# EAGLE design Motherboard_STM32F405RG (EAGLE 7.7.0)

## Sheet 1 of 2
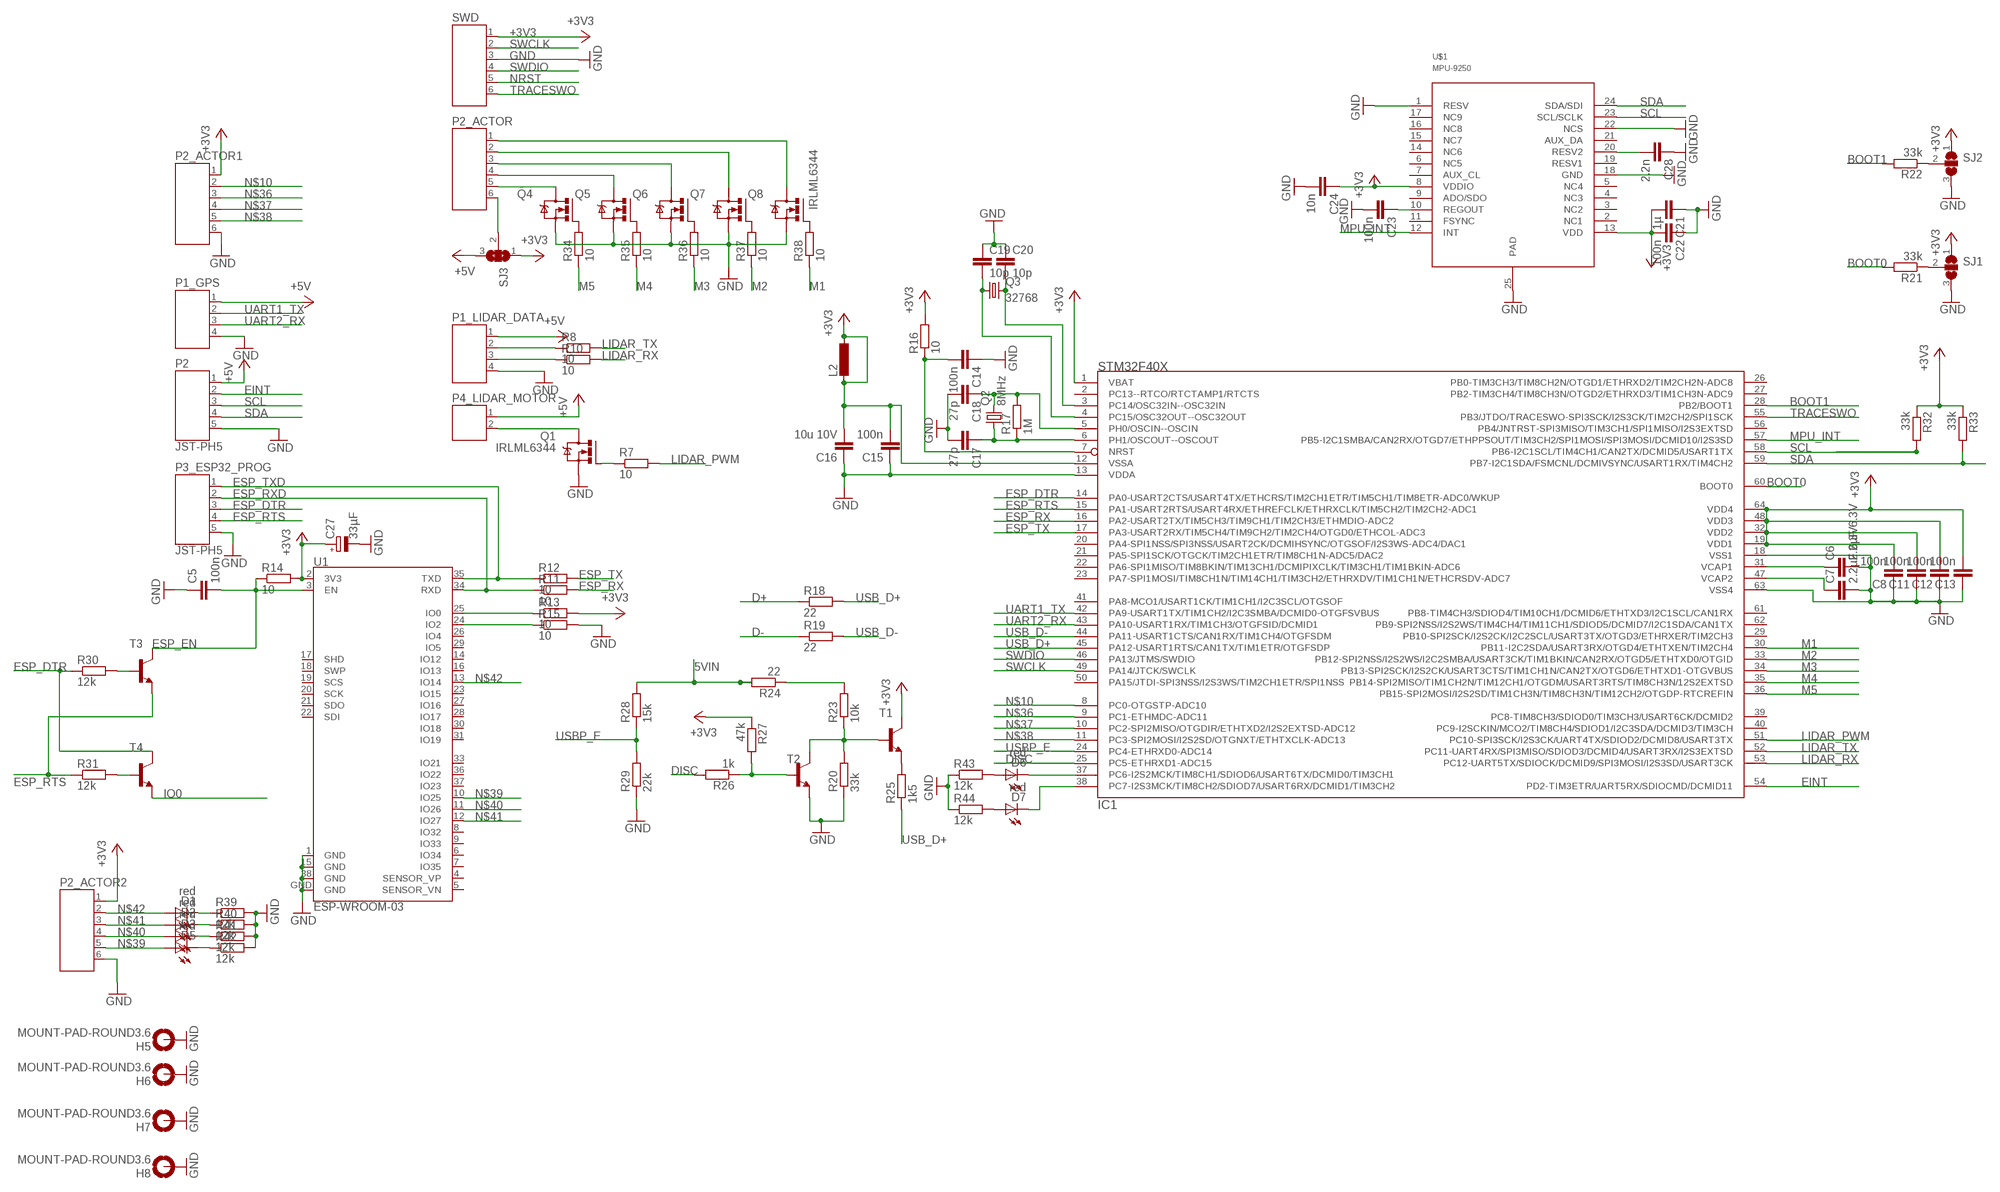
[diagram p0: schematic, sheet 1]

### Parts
C5  100n  C-EUC0603  [C0603]
C6  2.2µF 6.3V  C-EUC0603  [C0603]
C7  2.2µF 6.3V  C-EUC0603  [C0603]
C8  100n  C-EUC0603  [C0603]
C11  100n  C-EUC0603  [C0603]
C12  100n  C-EUC0603  [C0603]
C13  100n  C-EUC0603  [C0603]
C14  100n  C-EUC0603  [C0603]
C15  100n  C-EUC0603  [C0603]
C16  10u 10V  C-EUC1206  [C1206]
C17  27p  C-EUC0603  [C0603]
C18  27p  C-EUC0603  [C0603]
C19  10p  C-EUC0603  [C0603]
C20  10p  C-EUC0603  [C0603]
C21  1µ  C-EUC0603  [C0603]
C22  100n  C-EUC0603  [C0603]
C23  100n  C-EUC0603  [C0603]
C24  10n  C-EUC0603  [C0603]
C27  33µF  CPOL-EUA/3216-18W  [A/3216-18W]
C28  2.2n  C-EUC0603  [C0603]
D1  red  LED0603  [LED-0603]
D2  red  LED0603  [LED-0603]
D3  red  LED0603  [LED-0603]
D5  red  LED0603  [LED-0603]
D6  red  LED0603  [LED-0603]
D7  red  LED0603  [LED-0603]
H5  MOUNT-PAD-ROUND3.6  [3,6-PAD]
H6  MOUNT-PAD-ROUND3.6  [3,6-PAD]
H7  MOUNT-PAD-ROUND3.6  [3,6-PAD]
H8  MOUNT-PAD-ROUND3.6  [3,6-PAD]
IC1  STM32F40X  [LQFP64]
L2  L-EUL1812  [L1812]
P1_GPS  JST-PH4  [JST-PH4]
P1_LIDAR_DATA  JST-PH4  [JST-PH4]
P2  JST-PH5  [JST-PH5]
P2_ACTOR  JST-PH6  [JST-PH6]
P2_ACTOR1  JST-PH6  [JST-PH6]
P2_ACTOR2  JST-PH6  [JST-PH6]
P3_ESP32_PROG  JST-PH5  [JST-PH5]
P4_LIDAR_MOTOR  JST-PH2  [JST-PH2]
Q1  IRLML6344  [SOT23]
Q2  8MHz  CRYSTALHC18U-V  [HC18U-V]
Q3  32768  CRYSTALTC38H  [TC38H]
Q4  IRLML6344  [SOT23]
Q5  IRLML6344  [SOT23]
Q6  IRLML6344  [SOT23]
Q7  IRLML6344  [SOT23]
Q8  IRLML6344  [SOT23]
R7  10  R-EU_R0603  [R0603]
R8  10  R-EU_R0603  [R0603]
R10  10  R-EU_R0603  [R0603]
R11  10  R-EU_R0603  [R0603]
R12  10  R-EU_R0603  [R0603]
R13  10  R-EU_R0603  [R0603]
R14  10  R-EU_R0603  [R0603]
R15  10  R-EU_R0603  [R0603]
R16  10  R-EU_R0603  [R0603]
R17  1M  R-EU_R0603  [R0603]
R18  22  R-EU_R0603  [R0603]
R19  22  R-EU_R0603  [R0603]
R20  33k  R-EU_R0603  [R0603]
R21  33k  R-EU_R0603  [R0603]
R22  33k  R-EU_R0603  [R0603]
R23  10k  R-EU_R0603  [R0603]
R24  22  R-EU_R0603  [R0603]
R25  1k5  R-EU_R0603  [R0603]
R26  1k  R-EU_R0603  [R0603]
R27  47k  R-EU_R0603  [R0603]
R28  15k  R-EU_R0603  [R0603]
R29  22k  R-EU_R0603  [R0603]
R30  12k  R-EU_R0603  [R0603]
R31  12k  R-EU_R0603  [R0603]
R32  33k  R-EU_R0603  [R0603]
R33  33k  R-EU_R0603  [R0603]
R34  10  R-EU_R0603  [R0603]
R35  10  R-EU_R0603  [R0603]
R36  10  R-EU_R0603  [R0603]
R37  10  R-EU_R0603  [R0603]
R38  10  R-EU_R0603  [R0603]
R39  12k  R-EU_R0603  [R0603]
R40  12k  R-EU_R0603  [R0603]
R41  12k  R-EU_R0603  [R0603]
R42  12k  R-EU_R0603  [R0603]
R43  12k  R-EU_R0603  [R0603]
R44  12k  R-EU_R0603  [R0603]
SJ1  SJ2W  [SJ_2]
SJ2  SJ2W  [SJ_2]
SJ3  SJ2W  [SJ_2]
SWD  JST-PH6  [JST-PH6]
T1  BC817-16-NPN-SOT23-BEC  [SOT23-BEC]
T2  BC817-16-NPN-SOT23-BEC  [SOT23-BEC]
T3  BC817-16-NPN-SOT23-BEC  [SOT23-BEC]
T4  BC817-16-NPN-SOT23-BEC  [SOT23-BEC]
U1  ESP-WROOM-03  [ESP-WROOM-03]
U$1  MPU-9250  [LEAD-QFN24]

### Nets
5VIN: R24.2 R28.2 ; also sheet 2
+3V3: C8.2 C11.2 C12.2 C13.2 C15.2 C16.2 C21.2 C22.2 C24.1 C27.+ IC1.1(VBAT) IC1.12(VSSA) IC1.19(VDD1) IC1.32(VDD2) IC1.48(VDD3) IC1.64(VDD4) L2.1 L2.2 P2_ACTOR1.1 P2_ACTOR2.1 R13.2 R14.2 R16.2 R27.1 R32.1 R33.1 SJ1.1 SJ2.1 SJ3.1 SWD.1 T1.C U1.2(3V3) U$1.8(VDDIO) U$1.13(VDD) ; also sheet 2
+5V: P1_GPS.1 P1_LIDAR_DATA.1 P2.1 P4_LIDAR_MOTOR.1 SJ3.3 ; also sheet 2
BOOT0: IC1.60(BOOT0) R21.2
BOOT1: IC1.28(PB2/BOOT1) R22.2
D+: R18.1 ; also sheet 2
D-: R19.1 ; also sheet 2
DISC: IC1.25(PC5-ETHRXD1-ADC15) R26.2
EINT: IC1.54(PD2-TIM3ETR/UART5RX/SDIOCMD/DCMID11) P2.2
ESP_DTR: IC1.14(PA0-USART2CTS/USART4TX/ETHCRS/TIM2CH1ETR/TIM5CH1/TIM8ETR-ADC0/WKUP) P3_ESP32_PROG.3 R30.1 T4.C
ESP_EN: C5.2 R14.1 T3.C U1.3(EN)
ESP_RTS: IC1.15(PA1-USART2RTS/USART4RX/ETHREFCLK/ETHRXCLK/TIM5CH2/TIM2CH2-ADC1) P3_ESP32_PROG.4 R31.1 T3.E
ESP_RX: IC1.16(PA2-USART2TX/TIM5CH3/TIM9CH1/TIM2CH3/ETHMDIO-ADC2) R11.2
ESP_RXD: P3_ESP32_PROG.2 R11.1 U1.34(RXD)
ESP_TX: IC1.17(PA3-USART2RX/TIM5CH4/TIM9CH2/TIM2CH4/OTGD0/ETHCOL-ADC3) R12.2
ESP_TXD: P3_ESP32_PROG.1 R12.1 U1.35(TXD)
GND: C5.1 C6.2 C7.2 C8.1 C11.1 C12.1 C13.1 C14.1 C15.1 C16.1 C17.2 C18.2 C19.1 C20.1 C21.1 C22.1 C23.2 C24.2 C27.- C28.1 H5.B3,6(MOUNT) H6.B3,6(MOUNT) H7.B3,6(MOUNT) H8.B3,6(MOUNT) IC1.13(VDDA) IC1.18(VSS1) IC1.63(VSS4) P1_GPS.4 P1_LIDAR_DATA.4 P2.5 P2_ACTOR1.6 P2_ACTOR2.6 P3_ESP32_PROG.5 Q1.2(S) Q4.2(S) Q5.2(S) Q6.2(S) Q7.2(S) Q8.2(S) R15.2 R20.1 R29.1 R39.2 R40.2 R41.2 R42.2 R43.1 R44.1 SJ1.3 SJ2.3 SWD.3 T2.E U1.1(GND) U1.15(GND) U1.38(GND) U1.GND U$1.1(RESV) U$1.18(GND) U$1.22(NCS) U$1.25(PAD) ; also sheet 2
IO0: R13.1 T4.E U1.25(IO0)
IO2: R15.1 U1.24(IO2)
LIDAR_PWM: IC1.51(PC10-SPI3SCK/I2S3CK/UART4TX/SDIOD2/DCMID8/USART3TX) R7.2
LIDAR_RX: IC1.53(PC12-UART5TX/SDIOCK/DCMID9/SPI3MOSI/I2S3SD/USART3CK) R10.2
LIDAR_TX: IC1.52(PC11-UART4RX/SPI3MISO/SDIOD3/DCMID4/USART3RX/I2S3EXTSD) R8.2
M1: IC1.30(PB11-I2C2SDA/USART3RX/OTGD4/ETHTXEN/TIM2CH4) R38.1
M2: IC1.33(PB12-SPI2NSS/I2S2WS/I2C2SMBA/USART3CK/TIM1BKIN/CAN2RX/OTGD5/ETHTXD0/OTGID) R37.1
M3: IC1.34(PB13-SPI2SCK/I2S2CK/USART3CTS/TIM1CH1N/CAN2TX/OTGD6/ETHTXD1-OTGVBUS) R36.1
M4: IC1.35(PB14-SPI2MISO/TIM1CH2N/TIM12CH1/OTGDM/USART3RTS/TIM8CH3N/12S2EXTSD) R35.1
M5: IC1.36(PB15-SPI2MOSI/I2S2SD/TIM1CH3N/TIM8CH3N/TIM12CH2/OTGDP-RTCREFIN) R34.1
MPU_INT: IC1.57(PB5-I2C1SMBA/CAN2RX/OTGD7/ETHPPSOUT/TIM3CH2/SPI1MOSI/SPI3MOSI/DCMID10/I2S3SD) U$1.12(INT)
N$3: C28.2 U$1.20(RESV2)
N$4: P4_LIDAR_MOTOR.2 Q1.3(D)
N$5: Q1.1(G) R7.1
N$6: P1_LIDAR_DATA.2 R8.1
N$7: P1_LIDAR_DATA.3 R10.1
N$9: C23.1 U$1.10(REGOUT)
N$10: IC1.8(PC0-OTGSTP-ADC10) P2_ACTOR1.2
N$12: P2_ACTOR.5 Q4.3(D)
N$13: R31.2 T4.B
N$15: P2_ACTOR.4 Q5.3(D)
N$16: C17.1 IC1.6(PH1/OSCOUT--OSCOUT) Q2.1 R17.1
N$17: P2_ACTOR.3 Q6.3(D)
N$18: P2_ACTOR.2 Q7.3(D)
N$19: C18.1 IC1.5(PH0/OSCIN--OSCIN) Q2.2 R17.2
N$20: C19.2 IC1.4(PC15/OSC32OUT--OSC32OUT) Q3.1
N$21: C20.2 IC1.3(PC14/OSC32IN--OSC32IN) Q3.2
N$22: R20.2 R23.1 T1.B T2.C
N$23: R21.1 SJ1.2
N$24: R22.1 SJ2.2
N$25: P2_ACTOR.1 Q8.3(D)
N$26: R25.2 T1.E
N$27: R23.2 R24.1
N$28: R26.1 R27.2 T2.B
N$29: R30.2 T3.B
N$30: P2_ACTOR.6 SJ3.2
N$31: Q4.1(G) R34.2
N$32: Q5.1(G) R35.2
N$33: Q6.1(G) R36.2
N$34: Q7.1(G) R37.2
N$35: Q8.1(G) R38.2
N$36: IC1.9(PC1-ETHMDC-ADC11) P2_ACTOR1.3
N$37: IC1.10(PC2-SPI2MISO/OTGDIR/ETHTXD2/I2S2EXTSD-ADC12) P2_ACTOR1.4
N$38: IC1.11(PC3-SPI2MOSI/I2S2SD/OTGNXT/ETHTXCLK-ADC13) P2_ACTOR1.5
N$39: D5.A P2_ACTOR2.5 U1.10(IO25)
N$40: D3.A P2_ACTOR2.4 U1.11(IO26)
N$41: D2.A P2_ACTOR2.3 U1.12(IO27)
N$42: D1.A P2_ACTOR2.2 U1.13(IO14)
N$43: D1.C R39.1
N$44: D2.C R40.1
N$45: D3.C R41.1
N$46: D5.C R42.1
N$48: D6.C IC1.37(PC6-I2S2MCK/TIM8CH1/SDIOD6/USART6TX/DCMID0/TIM3CH1)
N$49: D7.C IC1.38(PC7-I2S3MCK/TIM8CH2/SDIOD7/USART6RX/DCMID1/TIM3CH2)
N$50: D6.A R43.2
N$51: D7.A R44.2
NRST: C14.2 IC1.7(NRST) R16.1 SWD.5
SCL: IC1.58(PB6-I2C1SCL/TIM4CH1/CAN2TX/DCMID5/USART1TX) P2.3 R32.2 U$1.23(SCL/SCLK)
SDA: IC1.59(PB7-I2C1SDA/FSMCNL/DCMIVSYNC/USART1RX/TIM4CH2) P2.4 R33.2 U$1.24(SDA/SDI)
SWCLK: IC1.49(PA14/JTCK/SWCLK) SWD.2
SWDIO: IC1.46(PA13/JTMS/SWDIO) SWD.4
TRACESWO: IC1.55(PB3/JTDO/TRACESWO-SPI3SCK/I2S3CK/TIM2CH2/SPI1SCK) SWD.6
UART1_TX: IC1.42(PA9-USART1TX/TIM1CH2/I2C3SMBA/DCMID0-OTGFSVBUS) P1_GPS.2
UART2_RX: IC1.43(PA10-USART1RX/TIM1CH3/OTGFSID/DCMID1) P1_GPS.3
USB_D+: IC1.45(PA12-USART1RTS/CAN1TX/TIM1ETR/OTGFSDP) R18.2 R25.1
USB_D-: IC1.44(PA11-USART1CTS/CAN1RX/TIM1CH4/OTGFSDM) R19.2
USBP_E: IC1.24(PC4-ETHRXD0-ADC14) R28.1 R29.2
VCAP1: C6.1 IC1.31(VCAP1)
VCAP2: C7.1 IC1.47(VCAP2)
Unconnected: IC1.2(PC13--RTCO/RTCTAMP1/RTCTS) IC1.20(PA4-SPI1NSS/SPI3NSS/USART2CK/DCMIHSYNC/OTGSOF/I2S3WS-ADC4/DAC1) IC1.21(PA5-SPI1SCK/OTGCK/TIM2CH1ETR/TIM8CH1N-ADC5/DAC2) IC1.22(PA6-SPI1MISO/TIM8BKIN/TIM13CH1/DCMIPIXCLK/TIM3CH1/TIM1BKIN-ADC6) IC1.23(PA7-SPI1MOSI/TIM8CH1N/TIM14CH1/TIM3CH2/ETHRXDV/TIM1CH1N/ETHCRSDV-ADC7) IC1.26(PB0-TIM3CH3/TIM8CH2N/OTGD1/ETHRXD2/TIM2CH2N-ADC8) IC1.27(PB2-TIM3CH4/TIM8CH3N/OTGD2/ETHRXD3/TIM1CH3N-ADC9) IC1.29(PB10-SPI2SCK/I2S2CK/I2C2SCL/USART3TX/OTGD3/ETHRXER/TIM2CH3) IC1.39(PC8-TIM8CH3/SDIOD0/TIM3CH3/USART6CK/DCMID2) IC1.40(PC9-I2SCKIN/MCO2/TIM8CH4/SDIOD1/I2C3SDA/DCMID3/TIM3CH) IC1.41(PA8-MCO1/USART1CK/TIM1CH1/I2C3SCL/OTGSOF) IC1.50(PA15/JTDI-SPI3NSS/I2S3WS/TIM2CH1ETR/SPI1NSS) IC1.56(PB4/JNTRST-SPI3MISO/TIM3CH1/SPI1MISO/I2S3EXTSD) IC1.61(PB8-TIM4CH3/SDIOD4/TIM10CH1/DCMID6/ETHTXD3/I2C1SCL/CAN1RX) IC1.62(PB9-SPI2NSS/I2S2WS/TIM4CH4/TIM11CH1/SDIOD5/DCMID7/I2C1SDA/CAN1TX) U1.4(SENSOR_VP) U1.5(SENSOR_VN) U1.6(IO34) U1.7(IO35) U1.8(IO32) U1.9(IO33) U1.14(IO12) U1.16(IO13) U1.17(SHD) U1.18(SWP) U1.19(SCS) U1.20(SCK) U1.21(SDO) U1.22(SDI) U1.23(IO15) U1.26(IO4) U1.27(IO16) U1.28(IO17) U1.29(IO5) U1.30(IO18) U1.31(IO19) U1.33(IO21) U1.36(IO22) U1.37(IO23) U$1.2(NC1) U$1.3(NC2) U$1.4(NC3) U$1.5(NC4) U$1.6(NC5) U$1.7(AUX_CL) U$1.9(ADO/SDO) U$1.11(FSYNC) U$1.14(NC6) U$1.15(NC7) U$1.16(NC8) U$1.17(NC9) U$1.19(RESV1) U$1.21(AUX_DA)

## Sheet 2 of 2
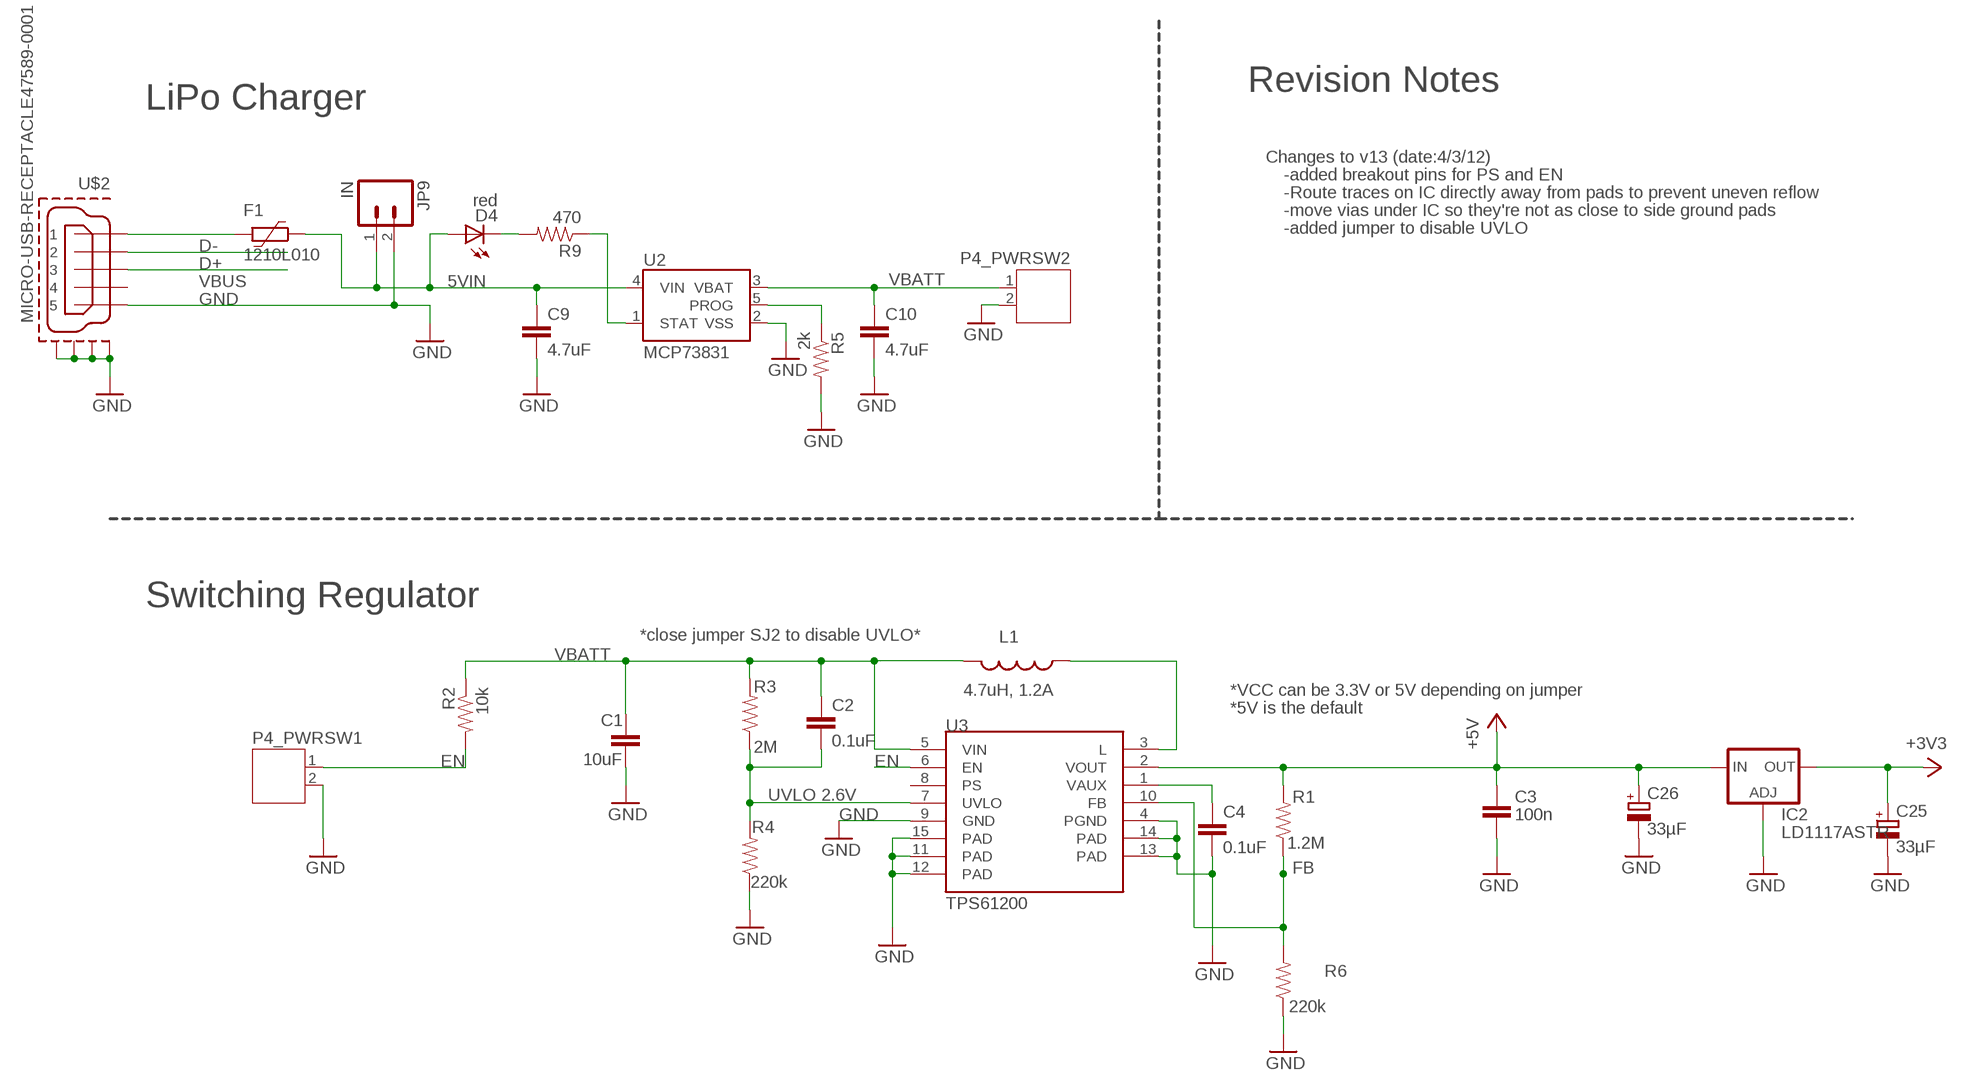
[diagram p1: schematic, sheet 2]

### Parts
C1  10uF  CAP1206  [1206]
C2  0.1uF  CAP0603-CAP  [0603-CAP]
C3  100n  CAP0805  [0805]
C4  0.1uF  CAP0603-CAP  [0603-CAP]
C9  4.7uF  CAP0603-CAP  [0603-CAP]
C10  4.7uF  CAP0603-CAP  [0603-CAP]
C25  33µF  CPOL-EUA/3216-18W  [A/3216-18W]
C26  33µF  CPOL-EUA/3216-18W  [A/3216-18W]
D4  red  LED0603  [LED-0603]
F1  1210L010  [1210L]
IC2  LD1117ASTR  LD117ASTR  [SOT223]
JP9  IN  M02PTH  [1X02]
L1  4.7uH, 1.2A  INDUCTOR.  [CDRH2D09]
P4_PWRSW1  JST-PH2  [JST-PH2]
P4_PWRSW2  JST-PH2  [JST-PH2]
R1  1.2M  RESISTOR0603-RES  [0603-RES]
R2  10k  RESISTOR0603-RES  [0603-RES]
R3  2M  RESISTOR0603-RES  [0603-RES]
R4  220k  RESISTOR0603-RES  [0603-RES]
R5  2k  RESISTOR0603-RES  [0603-RES]
R6  220k  RESISTOR0603-RES  [0603-RES]
R9  470  RESISTOR0603-RES  [0603-RES]
U2  MCP73831  [SOT23-5]
U3  TPS61200  [QFN-10_PAD]
U$2  MICRO-USB-RECEPTACLE47589-0001  [47589-0001]

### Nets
5VIN: C9.1 D4.A F1.1 JP9.1 U2.4(VIN) ; also sheet 1
+3V3: C25.+ IC2.2(OUT) IC2.4(OUT) ; also sheet 1
+5V: C3.1 C26.+ IC2.3(IN) R1.2 U3.2(VOUT) ; also sheet 1
D+: U$2.3 ; also sheet 1
D-: U$2.2 ; also sheet 1
EN: P4_PWRSW1.1 R2.2 U3.6(EN)
FB: R1.1 R6.2 U3.10(FB)
GND: C1.2 C3.2 C4.2 C9.2 C10.2 C25.- C26.- IC2.1(ADJ) JP9.2 P4_PWRSW1.2 P4_PWRSW2.2 R4.1 R5.2 R6.1 U2.2(VSS) U3.4(PGND) U3.9(GND) U3.11(PAD) U3.12(PAD) U3.13(PAD) U3.14(PAD) U3.15(PAD) U$2.5 U$2.CASING1(GND1) U$2.CASING2(GND2) U$2.CASING3(GND3) U$2.CASING4(GND4) ; also sheet 1
N$1: C4.1 U3.1(VAUX)
N$2: L1.P$1 U3.3(L)
N$8: D4.C R9.2
N$11: R5.1 U2.5(PROG)
N$14: R9.1 U2.1(STAT)
UVLO: C2.2 R3.1 R4.2 U3.7(UVLO)
VBATT: C1.1 C2.1 C10.1 L1.P$2 P4_PWRSW2.1 R2.1 R3.2 U2.3(VBAT) U3.5(VIN)
VBUS: F1.2 U$2.1
Unconnected: U3.8(PS) U$2.4

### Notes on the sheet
- Revision Notes
- LiPo Charger
- Changes to v13 (date:4/3/12)
- -added breakout pins for PS and EN
- -Route traces on IC directly away from pads to prevent uneven reflow
- -move vias under IC so they're not as close to side ground pads
- -added jumper to disable UVLO
- Switching Regulator
- *close jumper SJ2 to disable UVLO*
- *VCC can be 3.3V or 5V depending on jumper
- *5V is the default
- UVLO 2.6V

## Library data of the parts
C1 = CH_passive:CAP: Capacitor; MF: KEMET; MPN: C1206C106K8RACTU; OC_FARNELL: 1288264
C2 C4 = SparkFun:CAP: Capacitor; MF: YAGEO (PHYCOMP); MPN: CC0603MRY5V9BB104; OC_FARNELL: 431989
C3 = CH_passive:CAP: Capacitor; MF: KEMET; MPN: C0603C104K5RACTU; OC_FARNELL: 1288255
C5 C8 C11-C15 C22 C23 = rcl:C-EU: CAPACITOR, European symbol; MF: KEMET; MPN: C0603C104K5RACTU; OC_FARNELL: 1288255
C6 C7 = rcl:C-EU: CAPACITOR, European symbol; MF: KEMET; MPN: C0603C225K9PACTU; OC_FARNELL: 1288257
C9 C10 = SparkFun:CAP: Capacitor; MF: KEMET; MPN: C0603C475K8PACTU; OC_FARNELL: 1572625
C16 = rcl:C-EU: CAPACITOR, European symbol; MF: KEMET; MPN: C1206C106K8RACTU; OC_FARNELL: 1288264
C17 C18 = rcl:C-EU: CAPACITOR, European symbol; MF: YAGEO (PHYCOMP); MPN: CC0603JRNPO9BN270; OC_FARNELL: 722017
C19 C20 = rcl:C-EU: CAPACITOR, European symbol; MF: AVX; MPN: 06035A102JAT2A; OC_FARNELL: 317202
C21 = rcl:C-EU: CAPACITOR, European symbol; MF: AVX; MPN: 0603YC105KAT2A; OC_FARNELL: 1658870
C24 = rcl:C-EU: CAPACITOR, European symbol; MF: YAGEO (PHYCOMP); MPN: CC0603KRX7R9BB103; OC_FARNELL: 722236
C25-C27 = rcl:CPOL-EU: POLARIZED CAPACITOR, European symbol; MF: AVX; MPN: TPSA336M006R0600; OC_FARNELL: 2333095
C28 = rcl:C-EU: CAPACITOR, European symbol; MF: YAGEO (PHYCOMP); MPN: CC0603KRX7R9BB222; OC_FARNELL: 722194
D1-D7 = SparkFun:LED: LEDs; MF: OSRAM; MPN: LSQ976-Z; OC_FARNELL: 1226390
F1 = polyfuse-smd_10:?: Polyfuse Resettable PTC; MF: LITTELFUSE; MPN: 1210L010WR; OC_FARNELL: 1822206; OC_NEWARK: 18M4781
H5-H8 = holes_new:MOUNT-PAD-ROUND: MOUNTING PAD, round; OC_FARNELL: unknown
IC1 = pel_stm32:STM32F40X; MF: STMICROELECTRONICS; MPN: STM32F405RGT6; OC_FARNELL: 2064363
IC2 = v-reg:LD117A?*: Low drop fixed and adjustable positive voltage regulators 1 A Source: http://www.st.com/stonline/products/literature/ds/7194/ld1117axx.pdf; MF: ON SEMICONDUCTOR; MPN: NCP1117ST33T3G; OC_FARNELL: 1652366
JP9 = SparkFun:M02: Header 2; MF: JST (JAPAN SOLDERLESS TERMINALS); MPN: B2B-PH-K-S(LF)(SN); OC_FARNELL: 9491856
L1 = SparkFun:INDUCTOR: Inductors; MF: MURATA; MPN: LQH3NPN4R7MJ0L; OC_FARNELL: 2219271
L2 = rcl:L-EU: INDUCTOR, European symbol; OC_FARNELL: unknown
P1_GPS P1_LIDAR_DATA = jst-ph:JST-PH4; MF: JST (JAPAN SOLDERLESS TERMINALS); MPN: B4B-PH-K-S(LF)(SN); OC_FARNELL: 9492437
P2 P3_ESP32_PROG = jst-ph:JST-PH5; MF: JST (JAPAN SOLDERLESS TERMINALS); MPN: B5B-PH-K-S(LF)(SN); OC_FARNELL: 9492445
P2_ACTOR P2_ACTOR1 P2_ACTOR2 SWD = jst-ph:JST-PH6; MF: JST (JAPAN SOLDERLESS TERMINALS); MPN: B6B-PH-K-S(LF)(SN); OC_FARNELL: 9492453
P4_LIDAR_MOTOR P4_PWRSW1 P4_PWRSW2 = jst-ph:JST-PH2; MF: JST (JAPAN SOLDERLESS TERMINALS); MPN: B2B-PH-K-S(LF)(SN); OC_FARNELL: 9491856
Q1 Q4-Q8 = myDBv7:IRLML6344; MF: INFINEON; MPN: IRLML6344TRPBF; OC_FARNELL: 1857299
Q2 = crystal:CRYSTAL: CRYSTAL; MF: MULTICOMP; MPN: HC49S-8-30-50-70-30-ATF; OC_FARNELL: 1666997; OC_NEWARK: unknown
Q3 = crystal:CRYSTAL: CRYSTAL; MF: CITIZEN FINETECH MIYOTA; MPN: CFS206 32.768KDZB-UB; OC_FARNELL: 1457085; OC_NEWARK: unknown
R1 = SparkFun:RESISTOR: Resistor; MF: MULTICOMP; MPN: MCMR06W2004FTL; OC_FARNELL: 2073340
R2 = SparkFun:RESISTOR: Resistor; MF: MULTICOMP; MPN: MCMR06X1002FTL; OC_FARNELL: 2073349
R3 = SparkFun:RESISTOR: Resistor; MF: KOA SPEER ELECTRONICS; MPN: RK73H1JTTD1204F; OC_FARNELL: 1811595
R4 R6 = SparkFun:RESISTOR: Resistor; MF: MULTICOMP; MPN: MCHP03W8F2203T5E; OC_FARNELL: 1576314
R5 = SparkFun:RESISTOR: Resistor; MF: YAGEO (PHYCOMP); MPN: RC0603FR-072K2L.; OC_FARNELL: 9238522
R7 R8 R10-R16 R34-R38 = rcl:R-EU_: RESISTOR, European symbol; MF: VISHAY; MPN: CRCW060310R0FKEA; OC_FARNELL: 1469751
R9 = SparkFun:RESISTOR: Resistor; MF: MULTICOMP; MPN: MCHP03W8F4700T5E; OC_FARNELL: 1576273
R17 = rcl:R-EU_: RESISTOR, European symbol; MF: VISHAY; MPN: CRCW06031M00FKEA; OC_FARNELL: 1469746
R18 R19 R24 = rcl:R-EU_: RESISTOR, European symbol; MF: VISHAY; MPN: CRCW060322R0FKEA; OC_FARNELL: 1469781
R20-R22 R32 R33 = rcl:R-EU_: RESISTOR, European symbol; MF: VISHAY; MPN: CRCW060333K0FKEA; OC_FARNELL: 1469801
R23 = rcl:R-EU_: RESISTOR, European symbol; MF: MULTICOMP; MPN: MCMR06X1002FTL; OC_FARNELL: 2073349
R25 = rcl:R-EU_: RESISTOR, European symbol; MF: MULTICOMP; MPN: MCMR06X1501FTL; OC_FARNELL: 2073391
R26 = rcl:R-EU_: RESISTOR, European symbol; MF: VISHAY; MPN: CRCW06031K00FKEA; OC_FARNELL: 1469740
R27 = rcl:R-EU_: RESISTOR, European symbol; MF: VISHAY; MPN: CRCW060347K0FKEA; OC_FARNELL: 1469811
R28 = rcl:R-EU_: RESISTOR, European symbol; MF: VISHAY; MPN: CRCW060315K0FKEA; OC_FARNELL: 1469758
R29 = rcl:R-EU_: RESISTOR, European symbol; MF: TE CONNECTIVITY / NEOHM; MPN: CPF0603F4K22C1; OC_FARNELL: 1527541
R30 R31 R39-R44 = rcl:R-EU_: RESISTOR, European symbol; MF: MULTICOMP; MPN: MC0063W060312K8; OC_FARNELL: 1170832
SJ1-SJ3 = jumper:SJ2W: SMD solder JUMPER; OC_FARNELL: unknown
T1-T4 = transistor:*-NPN-: NPN Transistror BF959 corrected 2008.03.06; MF: NEXPERIA; MPN: BC817,215; OC_FARNELL: 1081223
U1 = esp32:ESP-WROOM-03; OC_FARNELL: unknown
U2 = SparkFun:MCP73831: Microchip's MCP73831 Miniature single cell, fully integrated Li-Ion, Li-polymer charge management controller http://ww1.microchip.com/downloads/en/DeviceDoc/21984a.pdf; MF: MICROCHIP; MPN: MCP73831T-2ACI/OT; OC_FARNELL: 1332158
U3 = SparkFun:TPS61200: DC to DC Booster; MF: TEXAS INSTRUMENTS; MPN: TPS61200DRCT; OC_FARNELL: 1471238
U$1 = invensense:MPU-9250; MF: INVENSENSE; MPN: MPU-6050; OC_FARNELL: 1864742
U$2 = con-molex-usb:MICRO-USB-RECEPTACLE: MICRO USB RECEPTACLES Micro-USB Receptacles, SMT, Lead-Free from MOLEX. (C) 2014 Tomasz Boleslaw CEDRO, cederom@tlen.pl, http://www.tomek.cedro.info. Version 0.1 (2014-01-17): Initial release. Version 0.2 (2014-02-06): Updated 47589-0001 footprint pins/pads/milling. Following devices are included: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; MF: MOLEX; MPN: 47589-0001; OC_FARNELL: 1568023

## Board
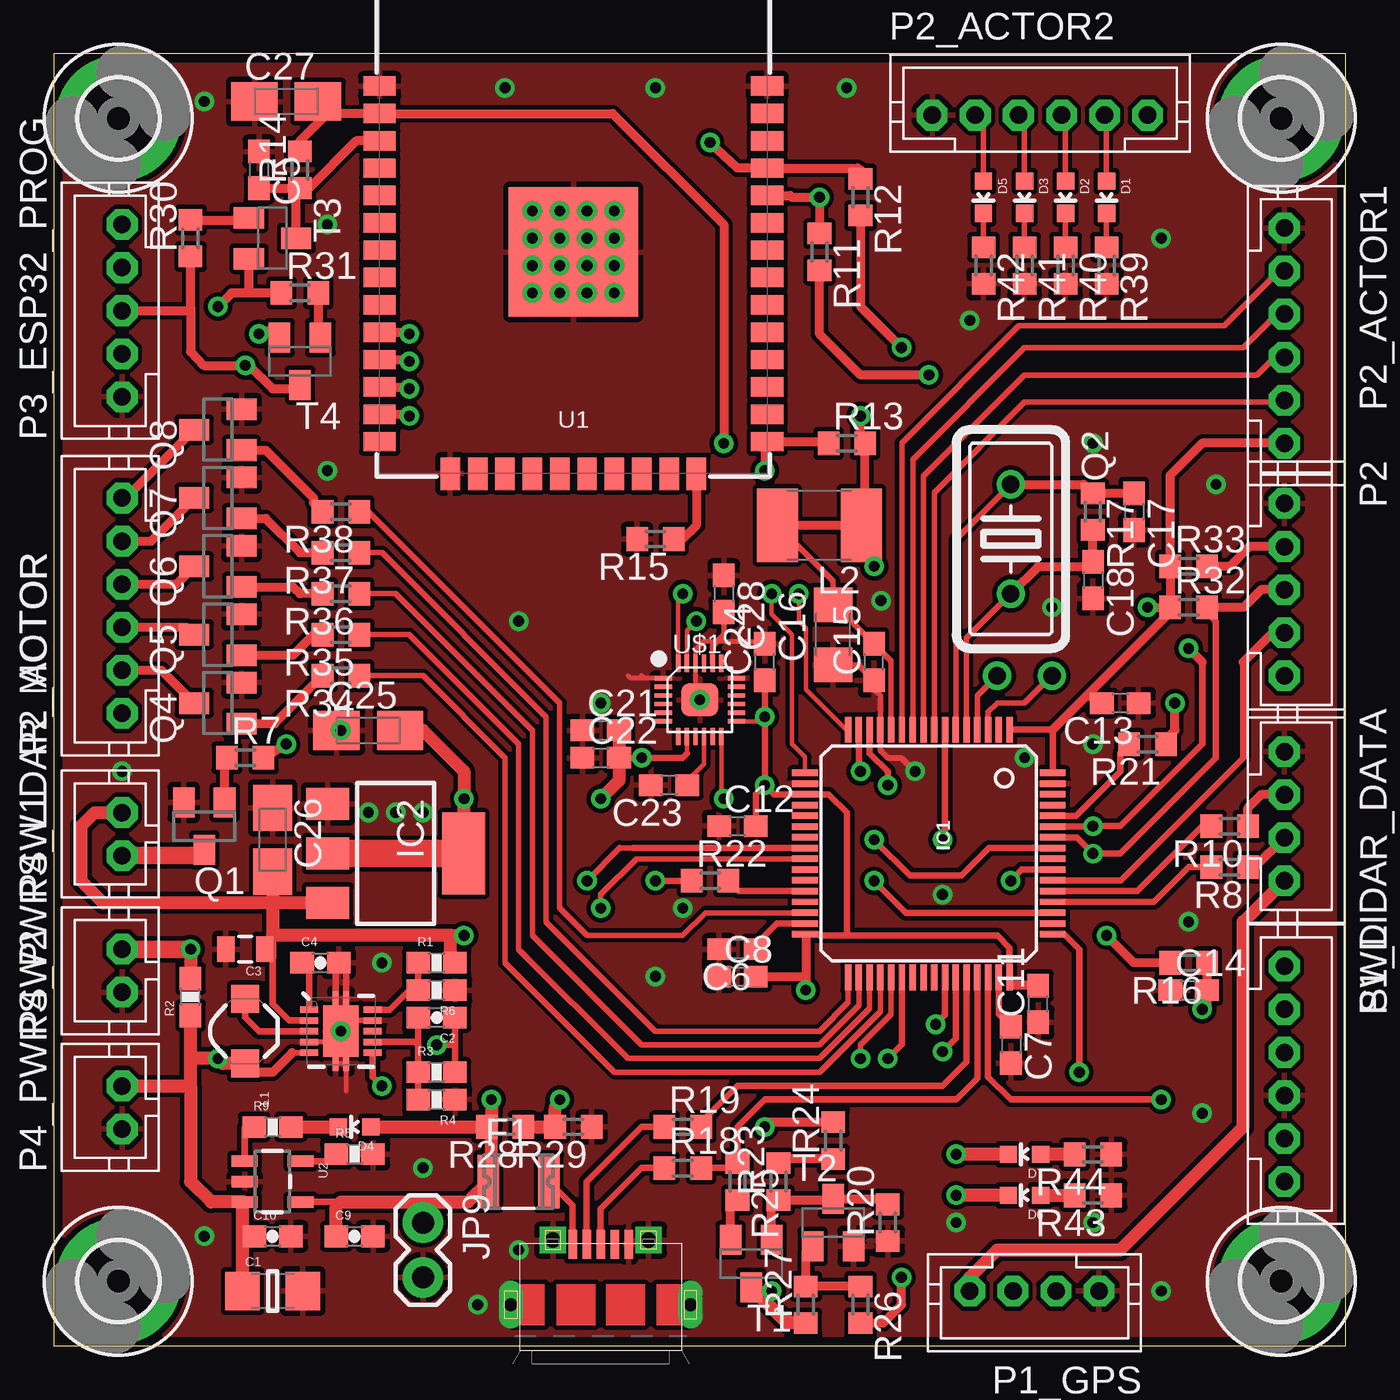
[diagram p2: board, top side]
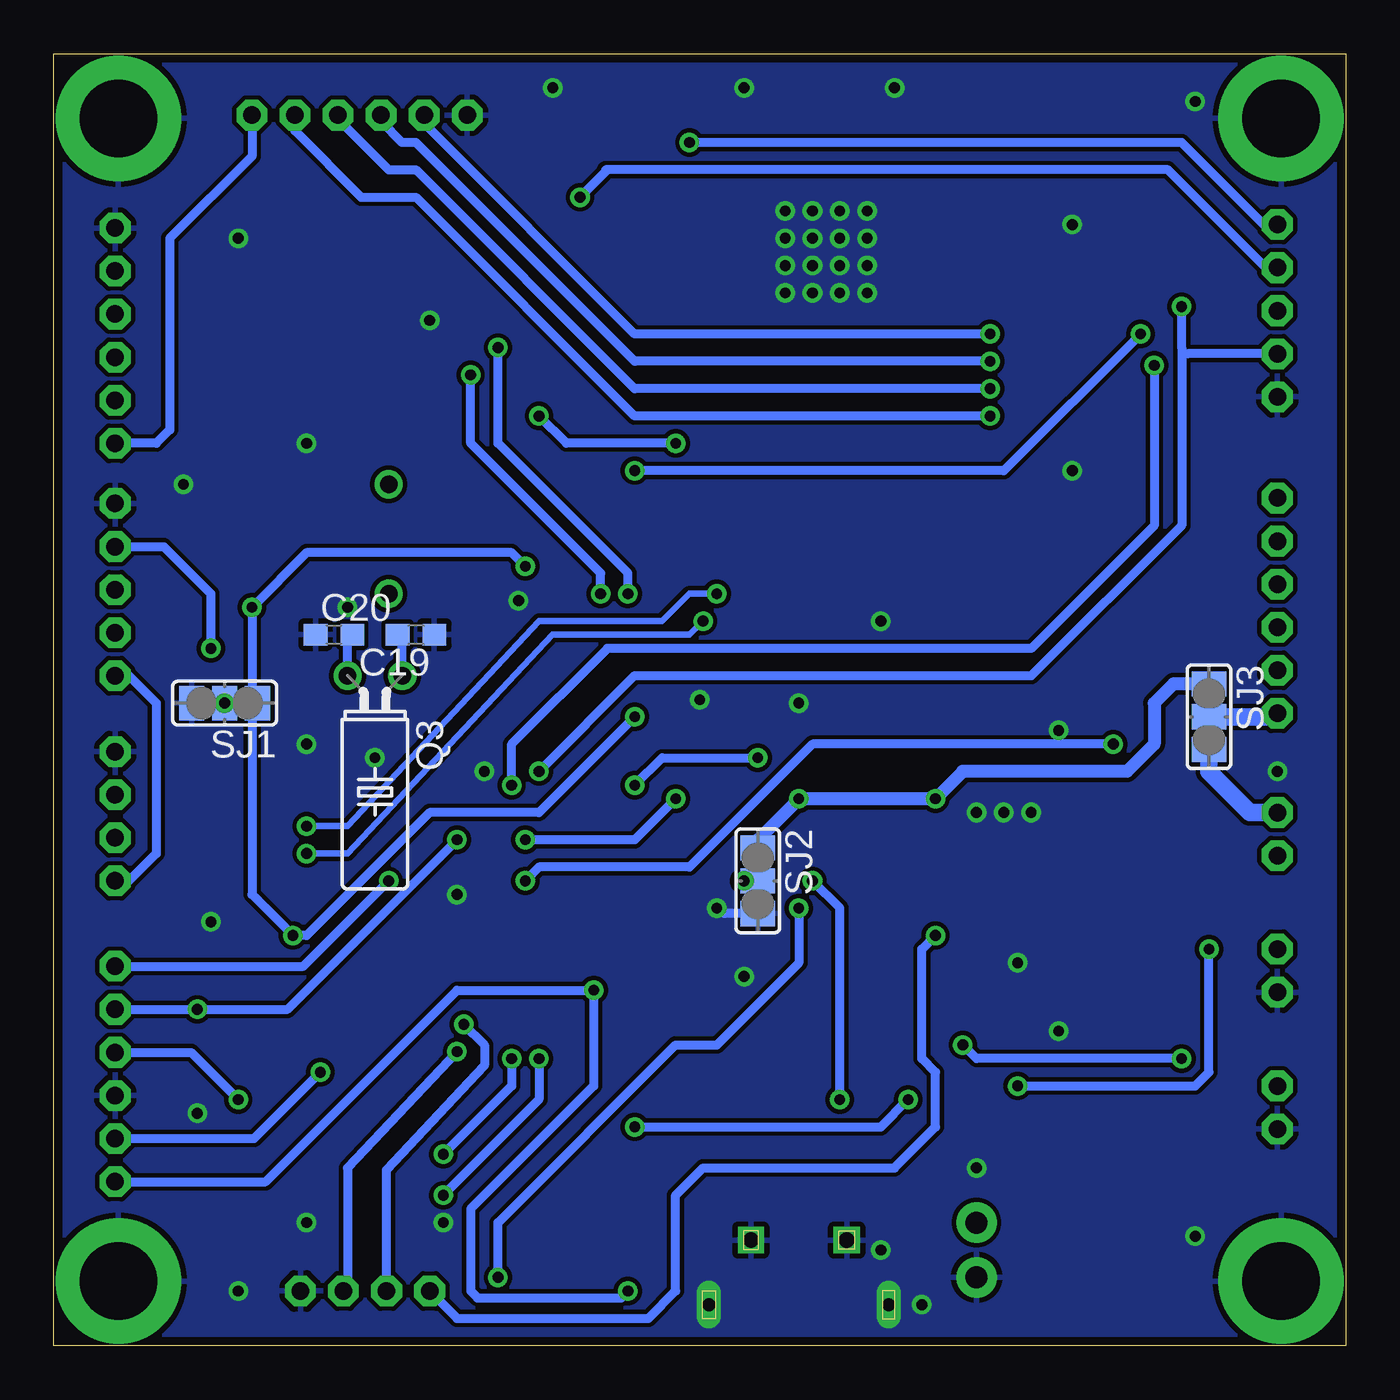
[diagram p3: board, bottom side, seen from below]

Size 60 x 60 mm. Coordinates in mm from the lower left corner, seen from the top.
Outline: 0,0 60,0 60,60 0,60 0,0
Copper layers (1*16): Top 0.035mm / dielectric 1.5mm / Bottom 0.035mm
Design rules "default *": minimum track width 10mil, minimum drill 0.6mm, track to track 8mil, track to pad 8mil, pad to pad 8mil, via to via 8mil, smd to smd 8mil, copper to edge 16mil, drill to drill 8mil, minimum pad ring 10mil, minimum via ring 8mil, stop-mask expansion 4mil, vias tented up to drill 0mil, thermal gap 10mil

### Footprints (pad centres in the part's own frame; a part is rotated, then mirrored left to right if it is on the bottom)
1206 = smd 1.6 x 1.8: 1 -1.4,0; 2 1.4,0
0603-CAP = smd 1.1 x 1: 1 -0.85,0; 2 0.85,0
0805 = smd 0.8 x 1.2: 1 -0.9,0; 2 0.9,0
C0603 = smd 1.1 x 1: 1 -0.85,0; 2 0.85,0
C1206 = smd 1.6 x 1.8: 1 -1.4,0; 2 1.4,0
A/3216-18W = smd 2.15 x 1.8: + 1.475,0; - -1.475,0
LED-0603 = smd 0.8 x 0.8: A 0,-0.75; C 0,0.75
1210L = smd 1 x 2.5: 1 -1.4,0; 2 1.4,0
3,6-PAD = drill 3.6 pad 5.842: B3,6 0,0
LQFP64 = smd 1.2 x 0.3: 1 -5.75,3.75; 2 -5.75,3.25; 3 -5.75,2.75; 4 -5.75,2.25; 5 -5.75,1.75; 6 -5.75,1.25; 7 -5.75,0.75; 8 -5.75,0.25; 9 -5.75,-0.25; 10 -5.75,-0.75; 11 -5.75,-1.25; 12 -5.75,-1.75; 13 -5.75,-2.25; 14 -5.75,-2.75; 15 -5.75,-3.25; 16 -5.75,-3.75; 33 5.75,-3.75; 34 5.75,-3.25; 35 5.75,-2.75; 36 5.75,-2.25; 37 5.75,-1.75; 38 5.75,-1.25; 39 5.75,-0.75; 40 5.75,-0.25; 41 5.75,0.25; 42 5.75,0.75; 43 5.75,1.25; 44 5.75,1.75; 45 5.75,2.25; 46 5.75,2.75; 47 5.75,3.25; 48 5.75,3.75 | smd 0.3 x 1.2: 17 -3.75,-5.75; 18 -3.25,-5.75; 19 -2.75,-5.75; 20 -2.25,-5.75; 21 -1.75,-5.75; 22 -1.25,-5.75; 23 -0.75,-5.75; 24 -0.25,-5.75; 25 0.25,-5.75; 26 0.75,-5.75; 27 1.25,-5.75; 28 1.75,-5.75; 29 2.25,-5.75; 30 2.75,-5.75; 31 3.25,-5.75; 32 3.75,-5.75; 49 3.75,5.75; 50 3.25,5.75; 51 2.75,5.75; 52 2.25,5.75; 53 1.75,5.75; 54 1.25,5.75; 55 0.75,5.75; 56 0.25,5.75; 57 -0.25,5.75; 58 -0.75,5.75; 59 -1.25,5.75; 60 -1.75,5.75; 61 -2.25,5.75; 62 -2.75,5.75; 63 -3.25,5.75; 64 -3.75,5.75
SOT223 = smd 1.5 x 2: 1 -2.3,-3.15; 2 0,-3.15; 3 2.3,-3.15 | smd 3.8 x 2: 4 0,3.15
1X02 = drill 1.016 pad 1.88: 1 0,0; 2 2.54,0
CDRH2D09 = smd 1.3 x 1.3: P$1 -1.5,0; P$2 1.5,0
L1812 = smd 1.9 x 3.4: 1 -1.95,0; 2 1.95,0
JST-PH4 = drill 0.813 pad 1.422 octagon: 1 0,0; 2 -2,0; 3 -4,0; 4 -6,0
JST-PH5 = drill 0.813 pad 1.422 octagon: 1 0,0; 2 -2,0; 3 -4,0; 4 -6,0; 5 -8,0
JST-PH6 = drill 0.813 pad 1.422 octagon: 1 0,0; 2 -2,0; 3 -4,0; 4 -6,0; 5 -8,0; 6 -10,0
JST-PH2 = drill 0.813 pad 1.422 octagon: 1 0,0; 2 -2,0
SOT23 = smd 1 x 1.4: 1 -0.95,-1.1; 2 0.95,-1.1; 3 0,1.1
HC18U-V = drill 0.813: 1 -2.54,0; 2 2.54,0
TC38H = drill 0.813: 1 -1.27,0; 2 1.27,0
0603-RES = smd 1.1 x 1: 1 -0.85,0; 2 0.85,0
R0603 = smd 1 x 1.1: 1 -0.85,0; 2 0.85,0
SJ_2 = smd 1.168 x 1.6: 1 -1.524,0; 2 0,0; 3 1.524,0
SOT23-BEC = smd 1 x 1.4: B -0.95,-1.1; C 0,1.1; E 0.95,-1.1
ESP-WROOM-03 = smd 0.9 x 1.5: 1 7.7,9; 2 6.43,9; 3 5.16,9; 4 3.89,9; 5 2.62,9; 6 1.35,9; 7 0.08,9; 8 -1.19,9; 9 -2.46,9; 10 -3.73,9; 11 -5,9; 12 -6.27,9; 13 -7.54,9; 14 -8.81,9; 25 -8.81,-9; 26 -7.54,-9; 27 -6.27,-9; 28 -5,-9; 29 -3.73,-9; 30 -2.46,-9; 31 -1.19,-9; 32 0.08,-9; 33 1.35,-9; 34 2.62,-9; 35 3.89,-9; 36 5.16,-9; 37 6.43,-9; 38 7.7,-9 | smd 1.5 x 0.9: 15 -10.3,5.715; 16 -10.3,4.445; 17 -10.3,3.175; 18 -10.3,1.905; 19 -10.3,0.635; 20 -10.3,-0.635; 21 -10.3,-1.905; 22 -10.3,-3.175; 23 -10.3,-4.445; 24 -10.3,-5.715 | smd 6 x 6: GND 0,0
SOT23-5 = smd 0.55 x 1.2: 1 -0.95,-1.3; 2 0,-1.3; 3 0.95,-1.3; 4 0.95,1.3; 5 -0.95,1.3
QFN-10_PAD = smd 0.297 x 0.85: 1 -1,-1.475; 2 -0.5,-1.475; 3 0,-1.475; 4 0.5,-1.475; 5 1,-1.475; 6 1,1.475; 7 0.5,1.475; 8 0,1.475; 9 -0.5,1.475; 10 -1,1.475 | smd 0.7 x 0.28: 11 -1.5,0.25; 12 -1.5,-0.25; 13 1.5,0.25; 14 1.5,-0.25 | smd 2.4 x 1.65: 15 0,0
LEAD-QFN24 = smd 0.8 x 0.2: 1 -1.7,1; 2 -1.7,0.6; 3 -1.7,0.2; 4 -1.7,-0.2; 5 -1.7,-0.6; 6 -1.7,-1; 13 1.7,-1; 14 1.7,-0.6; 15 1.7,-0.2; 16 1.7,0.2; 17 1.7,0.6; 18 1.7,1 | smd 0.2 x 0.8: 7 -1,-1.7; 8 -0.6,-1.7; 9 -0.2,-1.7; 10 0.2,-1.7; 11 0.6,-1.7; 12 1,-1.7; 19 1,1.7; 20 0.6,1.7; 21 0.2,1.7; 22 -0.2,1.7; 23 -0.6,1.7; 24 -1,1.7 | smd 1.7 x 1.54: 25 0,0
47589-0001 = smd 1.35 x 0.4: 1 2.8,1.3; 2 2.8,0.65; 3 2.8,0; 4 2.8,-0.65; 5 2.8,-1.3 | drill 0.6 pad 0.95 long: CASING1 0,4.175; CASING2 0,-4.175 | drill 0.7 pad 1.1 square: CASING3 3,2.225; CASING4 3,-2.225

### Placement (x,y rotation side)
C1  10.16,2.54 0 top
C2  17.78,15.24 180 top
C3  8.89,18.41 180 top
C4  12.38,17.78 0 top
C5  9.53,54.61 270 top
C6  31.75,18.41 180 top
C7  44.45,13.97 270 top
C8  31.75,17.14 0 top
C9  13.97,5.08 0 top
C10  10.16,5.08 0 top
C11  45.72,15.88 90 top
C12  31.75,24.13 0 top
C13  49.53,29.84 180 top
C14  52.7,16.51 0 top
C15  38.1,31.75 90 top
C16  36.2,33.02 90 top
C17  50.16,38.73 270 top
C18  48.26,35.56 270 top
C19  43.18,33.02 180 bottom
C20  46.99,33.02 0 bottom
C21  25.4,28.57 0 top
C22  25.4,27.3 0 top
C23  28.57,26.04 180 top
C24  33.02,31.75 90 top
C25  14.61,28.57 0 top
C26  10.16,23.5 270 top
C27  10.79,57.78 0 top
C28  31.11,34.92 270 top
D1  48.9,53.34 180 top
D2  46.99,53.34 180 top
D3  45.09,53.34 180 top
D4  13.97,10.16 90 top
D5  43.18,53.34 180 top
D6  45.09,6.99 90 top
D7  45.09,8.89 90 top
F1  21.59,7.62 0 top
H5  3,3 0 top
H6  57,3 0 top
H7  57,57 0 top
H8  3,57 0 top
IC1  40.64,22.86 270 top
IC2  15.88,22.86 270 top
JP9  17.14,5.71 270 top
L1  8.89,14.61 270 top
L2  35.56,38.1 180 top
P1_GPS  42.55,2.54 180 top
P1_LIDAR_DATA  57.15,21.59 270 top
P2  57.15,31.11 270 top
P2_ACTOR  3.17,39.37 90 top
P2_ACTOR1  57.15,41.91 270 top
P2_ACTOR2  50.8,57.15 0 top
P3_ESP32_PROG  3.17,52.07 90 top
P4_LIDAR_MOTOR  3.17,24.77 90 top
P4_PWRSW1  3.17,18.41 90 top
P4_PWRSW2  3.17,12.06 90 top
Q1  6.99,24.13 180 top
Q2  44.45,37.47 270 top
Q3  45.09,31.11 180 bottom
Q4  7.62,29.84 90 top
Q5  7.62,33.02 90 top
Q6  7.62,36.2 90 top
Q7  7.62,39.37 90 top
Q8  7.62,42.55 90 top
R1  17.78,17.78 0 top
R2  6.35,16.19 90 top
R3  17.78,12.7 0 top
R4  17.78,11.43 180 top
R5  13.97,8.89 0 top
R6  17.78,16.51 180 top
R7  8.89,27.3 0 top
R8  54.61,22.23 180 top
R9  10.16,10.16 0 top
R10  54.61,24.13 180 top
R11  35.56,50.8 270 top
R12  37.47,53.34 270 top
R13  36.83,41.91 0 top
R14  11.43,54.61 90 top
R15  27.94,37.47 180 top
R16  52.7,17.78 180 top
R17  48.26,38.73 270 top
R18  29.21,8.26 0 top
R19  29.21,10.16 0 top
R20  38.73,5.71 90 top
R21  50.8,27.94 180 top
R22  30.48,21.59 0 top
R23  33.66,7.62 90 top
R24  36.2,9.53 90 top
R25  31.75,7.62 270 top
R26  37.47,1.91 270 top
R27  34.92,1.91 90 top
R28  20.95,10.16 180 top
R29  24.13,10.16 180 top
R30  6.35,51.44 90 top
R31  11.43,48.9 0 top
R32  52.7,34.29 0 top
R33  52.7,36.2 0 top
R34  13.34,31.11 180 top
R35  13.34,33.02 180 top
R36  13.34,34.92 180 top
R37  13.34,36.83 180 top
R38  13.34,38.73 180 top
R39  48.9,50.16 270 top
R40  46.99,50.16 270 top
R41  45.09,50.16 270 top
R42  43.18,50.16 270 top
R43  48.26,6.99 180 top
R44  48.26,8.89 180 top
SJ1  52.07,29.84 180 bottom
SJ2  27.3,21.59 270 bottom
SJ3  6.35,29.21 270 bottom
SWD  57.15,7.62 270 top
T1  32.38,3.81 180 top
T2  36.2,5.71 0 top
T3  10.16,51.44 270 top
T4  11.43,45.72 180 top
U1  24.13,50.8 90 top
U2  10.16,7.62 270 top
U3  13.34,14.61 270 top
U$1  30,30 0 top
U$2  25.4,1.91 90 top

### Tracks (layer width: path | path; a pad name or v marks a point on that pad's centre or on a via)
5VIN  (via drill 0.5)
  Top 0.305: U2.4 13.34,6.67 13.12,6.46 | F1.1 20.19,7.75 20.32,8.26 | 20.32,10.16 R28.2 20.32,9.95
  Top 0.406: R24.2 33.23,10.38 v33.02,10.16
  Top 0.61: 13.34,6.67 17.14,6.67 | JP9.1 17.14,6.67 | D4.A R28.2 | v20.32,11.43 20.32,10.16 | 20.32,8.26 20.32,9.95 | 17.14,6.67 19.24,6.67 F1.1 | C9.1 13.12,6.46
  Bottom 0.406: v33.02,10.16 21.59,10.16 v20.32,11.43
+3V3  (via drill 0.5)
  Top 0.2: R13.2 37.47,41.91 | U$1.8 29.4,27.5 | U$1.13 32.81,29 v33.02,29.21 | 46.39,28.54 46.35,28.57 46.32,28.61 | R32.1 51.85,34.08 | 34.92,19.05 34.89,19.09 IC1.32 35.5,19.11 | 44.46,16.73 IC1.48 | C13.2 48.05,30.06 47.94,30.16
  Top 0.254: v38.1,36.2 38.1,37.51 L2.1 | IC1.12 38.89,31.81 C15.2 36.28,34.42 C16.2 36.2,35.52 L2.2
  Top 0.305: 19.05,22.86 IC2.4 | 29.4,27.5 29.21,27.3 v27.3,27.3 C22.2 | v33.02,26.04 33.45,25.61 IC1.19 35.98,25.61 36.83,24.77 36.83,19.05 | v33.02,26.04 v33.02,29.21 C24.1 | IC1.64 46.39,28.54 | IC1.1 46.32,28.61 | IC1.48 44.39,18.48 43.81,19.05 36.83,19.05 | 36.83,19.05 35.56,19.05 35.5,19.11 | C12.2 32.6,25.61 v33.02,26.04 | 32.22,2.54 T1.C
  Top 0.406: 51.85,34.08 47.94,30.16 46.35,28.57 | v31.11,41.91 31.11,52.07 25.95,57.23 U1.2 12.7,57.23 | 34.92,19.05 34.92,17.14 | 34.92,17.14 v34.92,16.51 | C11.2 44.46,16.73 | C8.2 34.92,17.14 | R16.2 50.16,17.78 v48.9,19.05 | P2_ACTOR1.1 53.34,41.91 51.85,40.42 R33.1 R32.1 v50.8,34.29 | v38.1,36.2 38.1,38.1 L2.1 | L2.1 L2.2 | 12.7,57.23 12.14,57.23 12.06,57.15 12.06,57.53 C27.+ | R14.2 11.43,55.96 12.7,57.23 | L2.1 37.68,38.1 R13.2 | 37.47,41.91 v37.47,43.18 | 32.22,2.54 v33.34,2.54
  Top 0.61: C21.2 C22.2 26.25,26.25 v25.4,25.4 | R27.1 34.04,1.05 T1.C | 19.05,22.86 v19.05,25.4 19.05,26.67 17.14,28.57 C25.+
  Top 1.27: IC2.2 IC2.4
  Bottom 0.2: v34.92,16.51 34.89,16.51 34.89,16.48 v34.92,16.51
  Bottom 0.305: SJ2.1 27.3,23.5 | SJ1.1 50.8,29.84
  Bottom 0.406: v33.02,26.04 31.75,27.3 v27.3,27.3 | v33.02,29.21 37.47,24.77 42.55,24.77 48.26,19.05 v48.9,19.05 50.8,20.95 50.8,29.84 v50.8,34.29 48.26,36.83 38.73,36.83 v38.1,36.2 | v31.11,41.91 36.2,41.91 v37.47,43.18 | SWD.1 50.16,7.62 41.27,16.51 v34.92,16.51 34.92,12.06 40.64,6.35 40.64,2.54 40.32,2.22 33.66,2.22 v33.34,2.54 | P2_ACTOR2.1 50.8,55.24 54.61,51.44 54.61,42.55 55.24,41.91 P2_ACTOR1.1
  Bottom 0.61: 27.3,23.5 v25.4,25.4 v19.05,25.4 17.78,26.67 10.16,26.67 8.89,27.94 8.89,29.84 8,30.73 SJ3.1
+5V  (via drill 0.5)
  Top 0.2: 18.43,19.04 18.43,19.07 | 19.04,19.07 v19.05,19.05
  Top 0.254: R1.2 18.41,17.78 18.43,17.8 | 18.43,19.04 18.41,19.05
  Top 0.305: U3.2 10.93,15.11 10.16,15.88 10.16,18.79 C3.1 10.19,18.02 10.19,19.05 10.16,19.05 | 10.16,20.32 10.4,20.56 10.16,20.56
  Top 0.406: 10.16,20.56 10.16,20.32
  Top 0.61: 10.16,20.32 10.16,19.05 | IC2.3 10.4,20.56 | P4_LIDAR_MOTOR.1 1.91,24.77 1.27,24.13 1.27,21.59 2.3,20.56 10.16,20.56 C26.+ | 18.43,17.8 18.43,19.04 | 18.41,19.05 10.19,19.05 | 18.43,19.07 19.04,19.07 | P1_GPS.1 42.55,3.17 43.81,4.45 49.53,4.45 55.24,10.16 55.24,19.68 P1_LIDAR_DATA.1
  Bottom 0.254: P2.1 56.52,31.11
  Bottom 0.406: P1_GPS.1 41.27,1.27 32.38,1.27 31.11,2.54 31.11,6.99 29.84,8.26 20.95,8.26 19.05,10.16 19.05,12.7 19.68,13.34 19.68,18.41 v19.05,19.05 | 56.52,31.11 55.24,29.84 55.24,22.86 56.52,21.59 P1_LIDAR_DATA.1
  Bottom 0.813: P4_LIDAR_MOTOR.1 4.45,24.77 6.35,26.67 SJ3.3
BOOT0
  Top 0.305: IC1.60 47.47,24.61 49.53,26.67 49.53,27.52 R21.2
BOOT1
  Top 0.305: IC1.28 31.81,21.11 R22.2
D+
  Top 0.305: R18.1 27.3,8.26 25.4,6.35 U$2.3
D-
  Top 0.305: R19.1 27.3,10.16 24.75,7.61 U$2.2
DISC  (via drill 0.5)
  Top 0.254: IC1.25 27.05,22.61 25.4,20.95 v25.4,20.32
  Top 0.406: R26.2 38.52,1.05 39.37,1.91 v39.37,3.17
  Bottom 0.406: v25.4,20.32 25.4,17.78 29.21,13.97 31.11,13.97 39.37,5.71 v39.37,3.17
EINT
  Top 0.305: IC1.54 49.55,21.61 55.24,27.3 55.24,31.75
  Top 0.406: P2.2 56.61,33.12 55.24,31.75
EN  (via drill 0.5)
  Top 0.305: U3.6 14.81,12.49 v15.24,12.06 | v6.35,18.41 6.37,18.41
  Top 0.61: 6.37,18.41 R2.2
  Top 0.813: P4_PWRSW1.1 v6.35,18.41
  Bottom 0.406: v15.24,12.06 6.99,12.06 6.35,12.7 v6.35,18.41
ESP_DTR  (via drill 0.5)
  Top 0.254: 6.16,48.07 6.35,48.26
  Top 0.305: IC1.14 37.89,27.52 38.73,26.67 v38.73,26.04
  Top 0.406: P3_ESP32_PROG.3 6.16,48.07 | v8.89,45.53 6.96,45.53 6.35,46.16 6.35,48.26 R30.1 | 9.06,45.7 v8.89,45.53 | v8.89,45.53 9.08,45.53 10.16,44.45 11.26,44.45 T4.C
  Bottom 0.2: v8.89,45.53 8.89,45.72
  Bottom 0.406: v38.73,26.04 38.73,27.94 34.29,32.38 14.61,32.38 8.89,38.1 v8.89,45.53
ESP_EN
  Top 0.406: U1.3 14.05,55.96 11.85,53.76 R14.1 | C5.2 R14.1 | T3.C 11.26,53.59 R14.1
ESP_RTS  (via drill 0.5)
  Top 0.305: IC1.15 37.39,26.75 v37.47,26.67
  Top 0.406: R31.1 8.89,48.9 | 8.89,48.9 8.26,48.9 v7.62,48.26 | T3.E 9.06,49.06 8.89,48.9
  Bottom 0.2: 7.33,46.07 7.62,46.35
  Bottom 0.406: v37.47,26.67 33.02,31.11 14.61,31.11 7.62,38.1 7.62,46.35 v7.62,48.26 | P3_ESP32_PROG.4 7.33,46.07
ESP_RX  (via drill 0.5)
  Top 0.2: IC1.16 36.8,28.61 34.92,30.48 34.92,33.34 34.61,33.66 v34.61,34.92
  Top 0.406: v40.64,45.09 37.47,45.09 35.56,46.99 R11.2
  Bottom 0.406: v34.61,34.92 34.61,35.88 40.64,41.91 v40.64,45.09
ESP_RXD  (via drill 0.5)
  Top 0.305: 35.77,53.34 v35.56,53.34
  Top 0.406: U1.34 34.21,53.42 34.29,53.34 v35.56,53.34 R11.1
  Bottom 0.254: 34.37,54.61 34.37,54.53
  Bottom 0.406: 34.37,54.61 8.26,54.61 3.71,50.07 P3_ESP32_PROG.2 | 34.37,54.53 v35.56,53.34
ESP_TX  (via drill 0.5)
  Top 0.2: IC1.17 34.89,27.34 34.29,27.94 34.29,33.02 33.34,33.97 v33.34,34.92
  Top 0.406: R12.2 37.47,48.26 v39.37,46.35
  Bottom 0.406: v33.34,34.92 33.34,35.88 39.37,41.91 v39.37,46.35
ESP_TXD  (via drill 0.5)
  Top 0.406: R12.1 37.47,54.61 37.33,54.69 U1.35 31.75,54.69 v30.48,55.88
  Bottom 0.406: P3_ESP32_PROG.1 3.81,52.07 7.62,55.88 v30.48,55.88
FB
  Top 0.305: U3.10 15.61,15.61 16.51,16.51 R6.2 R1.1
GND  (via drill 0.5)
  Top 0.2: U3.4 13.45,14.11 13.59,13.97 | U3.11 13.59,15.24 13.59,14.86 U3.15 | U3.14 U3.13 13.59,11.81 | 26.67,31.11 26.79,31 U$1.1 27.42,31 27.3,31.11 | U$1.25 29.8,30.2 U$1.22 29.8,32.34 30.16,32.7 32.92,32.7 C24.2
  Top 0.254: R44.1 48.9,8.89 | U1.GND v24.77,50.16 | U3.9 13.72,15.11 13.59,15.24 | C16.1 37.38,31.62 C15.1 38.1,30.48 38.39,30.19 IC1.13 38.39,27.65 38.73,27.3 39.37,27.3 v40.01,26.67
  Top 0.305: U3.11 13.59,17.55 C4.2 13.09,17.52 U3.12 | U3.13 13.59,13.97 13.59,14.61 U3.15
  Bottom 0.406: SJ2.3 28.83,20.07 v29.21,20.32
  other vias: 15.24,17.78 30,30 46.35,34.29 27.94,17.14 22.23,52.7 22.23,48.9 26.04,48.9 26.04,52.7 24.77,51.44 6.99,57.78 12.7,52.07 20.95,58.42 27.94,58.42 36.83,58.42 51.44,51.44 42.55,47.62 48.26,41.91 53.98,40.01 52.7,19.68 53.34,10.79 51.44,2.54 48.26,5.71 41.91,5.71 19.68,1.91 41.27,20.95 45.09,27.3 21.59,4.45 6.99,5.08 17.14,8.26 13.34,14.61 13.34,28.57 12.7,40.64 21.59,33.66 48.26,27.94 38.42,34.61 23.5,48.9 24.77,48.9 22.23,50.16 23.5,50.16 26.04,50.16 22.23,51.44 23.5,51.44 23.5,52.7 24.77,52.7 26.04,51.44 25.4,29.84 14.61,24.77 15.88,24.77 17.14,24.77 3.17,26.67
  pour Top: 0,60.33 60.33,60.33 60.33,0 0,0
  pour Bottom: 0,60.33 60.33,60.33 60.33,0 0,0
IO0  (via drill 0.5)
  Top 0.406: v33.02,40.64 33.02,41.91 32.94,41.99 U1.25 35.98,41.99 R13.1 | T4.E 10.48,47.31 v9.53,46.99
  Bottom 0.406: v9.53,46.99 15.88,40.64 v33.02,40.64
IO2
  Top 0.406: U1.24 29.84,38.1 29.21,37.47 R15.1
LIDAR_PWM  (via drill 0.5)
  Top 0.305: IC1.51 39.58,20.11 v38.1,21.59
  Top 0.406: R7.2 v10.79,27.94
  Bottom 0.406: v10.79,27.94 24.77,27.94 30.48,22.23 37.47,22.23 v38.1,21.59
LIDAR_RX
  Top 0.305: IC1.53 50.32,21.11 53.34,24.13 R10.2
LIDAR_TX
  Top 0.305: IC1.52 51.09,20.61 52.7,22.23 R8.2
M1
  Top 0.254: R38.1 14.61,38.73 23.5,29.84 23.5,20.32 24.77,19.05 29.21,19.05 30.27,20.11 IC1.30
M2
  Top 0.254: R37.1 15.24,36.83 22.86,29.21 22.86,19.68 27.94,14.61 35.56,14.61 36.89,15.94 IC1.33
M3
  Top 0.254: R36.1 15.88,34.92 22.23,28.57 22.23,19.05 27.3,13.97 35.56,13.97 37.39,15.8 IC1.34
M4
  Top 0.254: R35.1 16.51,33.02 21.59,27.94 21.59,18.41 26.67,13.34 35.56,13.34 37.89,15.66 IC1.35
M5
  Top 0.254: R34.1 17.14,31.11 20.95,27.3 20.95,17.78 26.04,12.7 35.56,12.7 38.39,15.53 IC1.36
MPU_INT  (via drill 0.5)
  Top 0.2: U$1.12 31,25.52 v31.11,25.4
  Top 0.305: IC1.57 43.43,23.11 42.16,21.84 39.76,21.84 v38.1,23.5
  Bottom 0.406: v31.11,25.4 33.02,23.5 v38.1,23.5
N$1
  Top 0.305: U3.1 11.86,17.59 C4.1
N$2
  Top 0.305: U3.3 9.53,14.61 8.89,15.24 L1.P$1
N$3
  Top 0.254: U$1.20 30.6,32.51 31.11,33.02 C28.2
N$4
  Top 0.305: 6.72,22.77 Q1.3
  Top 0.813: P4_LIDAR_MOTOR.2 6.72,22.77
N$5
  Top 0.2: 7.93,27.2 R7.1
  Top 0.406: Q1.1 7.93,27.2
N$6
  Top 0.406: R8.1 55.78,22.23 P1_LIDAR_DATA.2
N$7
  Top 0.406: P1_LIDAR_DATA.3 56.07,25.59 55.46,24.98 R10.1
N$8
  Top 0.61: R9.2 D4.C
N$9
  Top 0.2: U$1.10 30.2,27.02 29.21,26.04 29.21,25.82 C23.1
N$10
  Top 0.254: IC1.8 40.89,39.62 45.09,43.81 57.15,43.81 57.24,43.91 P2_ACTOR1.2
N$11
  Top 0.305: U2.5 13,8.57 R5.1
N$12
  Top 0.406: P2_ACTOR.5 5,31.37 Q4.3
N$13
  Top 0.406: R31.2 12.28,46.92 T4.B
N$14
  Top 0.305: U2.1 8.86,10.14 R9.1
N$15
  Top 0.406: P2_ACTOR.4 6.17,33.37 Q5.3
N$16
  Top 0.254: IC1.6 41.89,37.45 Q2.1
  Top 0.406: Q2.1 47.84,40.01 R17.1 C17.1
N$17
  Top 0.406: P2_ACTOR.3 5.7,35.37 Q6.3
N$18
  Top 0.406: P2_ACTOR.2 4.52,37.37 Q7.3
N$19
  Top 0.2: 48.48,36.2 C18.1
  Top 0.254: IC1.5 42.39,32.87 Q2.2
  Top 0.406: Q2.2 45.72,36.2 48.48,36.2 | C18.1 R17.2
N$20
  Top 0.254: IC1.4 42.89,30.19 Q3.1
  Bottom 0.2: 43.81,32.8 C19.2
  Bottom 0.406: Q3.1 43.81,32.8
N$21
  Top 0.254: IC1.3 43.39,29.42 43.81,29.84 45.09,29.84 Q3.2
  Bottom 0.2: 46.35,32.8 C20.2
  Bottom 0.406: Q3.2 46.35,32.8
N$22
  Top 0.305: 36.15,6.77 T2.C | 38.69,6.82 R20.2 | 33.34,6.45 R23.1
  Top 0.406: R23.1 36.15,6.77 | T2.C 38.69,6.82 | T1.B 33.34,6.45
N$23  (via drill 0.5)
  Top 0.406: R21.1 51.65,28.16 52.07,28.57 SJ1.2
  other vias: 52.07,29.84
N$24  (via drill 0.5)
  Top 0.305: R22.1 v27.94,21.59
  Bottom 0.305: SJ2.2 v27.94,21.59
N$25
  Top 0.406: 3.35,39.37 Q8.3
  Top 0.61: P2_ACTOR.1 3.35,39.37
N$26
  Top 0.305: 31.43,6.46 R25.2
  Top 0.406: T1.E 31.43,6.46
N$27
  Top 0.305: 33.86,8.68 R23.2
  Top 0.406: R24.1 33.86,8.68
N$28
  Top 0.305: 34.92,4.29 T2.B
  Top 0.406: 34.92,4.29 R27.2 R26.1
N$29
  Top 0.406: R30.2 8.96,52.28 T3.B
N$30
  Bottom 0.813: SJ3.2 3.33,29.21 P2_ACTOR.6
N$31
  Top 0.406: Q4.1 10.27,28.89 R34.2
N$32
  Top 0.305: 12.06,33.02 R35.2
  Top 0.406: Q5.1 11.11,32.07 12.06,33.02
N$33
  Top 0.406: Q6.1 11.11,35.24 11.43,34.92 R36.2
N$34
  Top 0.406: Q7.1 9.84,38.42 11.43,36.83 R37.2
N$35
  Top 0.406: Q8.1 9.84,41.59 12.06,39.37 12.06,39.16 R38.2
N$36
  Top 0.254: IC1.9 40.39,40.39 45.09,45.09 55.88,45.09 56.7,45.91 P2_ACTOR1.3
N$37
  Top 0.254: IC1.10 39.89,41.16 45.09,46.35 55.24,46.35 56.8,47.91 P2_ACTOR1.4
N$38
  Top 0.254: IC1.11 39.39,41.93 44.83,47.37 54.35,47.37 56.9,49.91 P2_ACTOR1.5
N$39  (via drill 0.5)
  Top 0.254: D5.A 43.18,56.77 P2_ACTOR2.5
  Top 0.406: U1.10 16.43,47.07 v16.51,46.99
  Bottom 0.254: 42.8,56.77 P2_ACTOR2.5
  Bottom 0.406: v16.51,46.99 33.02,46.99 42.8,56.77
N$40  (via drill 0.5)
  Top 0.254: D3.A 45.09,56.87 P2_ACTOR2.4
  Top 0.406: U1.11 16.43,45.8 v16.51,45.72
  Bottom 0.254: P2_ACTOR2.4 44.8,56.87
  Bottom 0.406: v16.51,45.72 33.02,45.72 43.18,55.88 43.81,55.88 44.8,56.87
N$41  (via drill 0.5)
  Top 0.254: D2.A 46.99,56.96 P2_ACTOR2.3
  Top 0.406: U1.12 16.43,44.53 v16.51,44.45
  Bottom 0.254: P2_ACTOR2.3 46.8,56.96
  Bottom 0.406: v16.51,44.45 33.02,44.45 43.18,54.61 44.45,54.61 46.8,56.96
N$42  (via drill 0.5)
  Top 0.254: D1.A 48.9,57.05 P2_ACTOR2.2
  Top 0.406: U1.13 16.43,43.26 v16.51,43.18
  Bottom 0.406: v16.51,43.18 33.02,43.18 43.18,53.34 45.72,53.34 48.8,56.42 P2_ACTOR2.2
N$43
  Top 0.254: D1.C R39.1
N$44
  Top 0.254: D2.C R40.1
N$45
  Top 0.254: D3.C R41.1
N$46
  Top 0.254: D5.C R42.1
N$48  (via drill 0.5)
  Top 0.254: IC1.37 38.89,15.39 37.47,13.97 v37.47,13.34
  Top 0.61: D6.C v41.91,6.99
  Bottom 0.406: v37.47,13.34 37.47,11.43 v41.91,6.99
N$49  (via drill 0.5)
  Top 0.305: IC1.38 39.39,13.99 v38.73,13.34
  Top 0.61: D7.C v41.91,8.89
  Bottom 0.406: v38.73,13.34 38.73,12.06 v41.91,8.89
N$50
  Top 0.61: D6.A R43.2
N$51
  Top 0.61: R44.2 D7.A
NRST  (via drill 0.5)
  Top 0.254: C14.2 R16.1 | 53.55,15.77 53.34,15.56 v53.34,15.62
  Top 0.305: IC1.7 41.39,23.61 v41.27,23.5
  Top 0.406: R16.1 53.55,15.77
  Bottom 0.406: SWD.5 v53.34,15.62 49.15,15.62 v41.27,23.5
SCL  (via drill 0.5)
  Top 0.2: U$1.23 29.4,33.21 v29.84,33.66
  Top 0.254: R32.2 53.55,34.05
  Top 0.305: IC1.58 47.51,23.61 v48.26,22.86 49.53,22.86 53.98,27.3 53.98,33.63 53.55,34.05
  Top 0.406: P2.3 56.07,35.12 55.24,34.29 R32.2
  Bottom 0.305: v29.84,33.66 30.48,33.02 36.83,33.02 46.35,22.86 v48.26,22.86
SDA  (via drill 0.5)
  Top 0.2: 46.37,24.12 46.35,24.13 | IC1.59 48.24,24.11 v48.26,24.13 v48.25,24.12 | U$1.24 29,34.72 v29.21,34.92
  Top 0.305: 53.34,31.75 53.34,27.94 49.53,24.13 v48.26,24.13 | 46.37,24.12 v48.25,24.12
  Top 0.406: 53.34,31.75 v52.7,32.38 | P2.4 55.53,37.12 54.61,36.2 R33.2
  Bottom 0.305: v29.21,34.92 30.48,34.92 31.75,33.66 37.47,33.66 46.35,24.13 v48.26,24.13
  Bottom 0.406: P2.4 54.9,37.12 52.7,34.92 v52.7,32.38
SWCLK  (via drill 0.5)
  Top 0.2: IC1.49 46.35,19.07 46.97,19.07
  Top 0.305: 46.97,19.07 47.62,18.41 v47.62,12.7
  Bottom 0.406: SWD.2 50.7,9.62 v47.62,12.7
SWDIO  (via drill 0.5)
  Top 0.305: IC1.46 43.39,12.49 44.45,11.43 v51.44,11.43
  Bottom 0.406: SWD.4 53.62,13.62 v51.44,11.43
TRACESWO  (via drill 0.5)
  Top 0.305: IC1.55 44.97,22.11 v44.45,21.59
  Bottom 0.406: SWD.6 48.42,17.62 v44.45,21.59
UART1_TX  (via drill 0.5)
  Top 0.305: IC1.42 41.39,15.36 v40.96,14.92
  Bottom 0.406: P1_GPS.2 44.55,8.16 40.01,13.02 40.01,13.97 v40.96,14.92
UART2_RX  (via drill 0.5)
  Top 0.305: IC1.43 41.89,14.27 v41.27,13.65
  Bottom 0.305: 46.35,2.73 P1_GPS.3
  Bottom 0.406: v41.27,13.65 46.35,8.26 46.35,2.73
USB_D+
  Top 0.305: IC1.45 42.89,12.41 41.91,11.43 33.02,11.43 31.75,10.16 R25.1 | 31.75,8.26 R25.1 | R18.2 30.06,8.47 30.48,8.26 31.54,8.26 R25.1
USB_D-
  Top 0.305: IC1.44 42.39,13.18 41.27,12.06 31.75,12.06 30.06,10.38 R19.2
USBP_E  (via drill 0.5)
  Top 0.254: 26.92,23.11 26.29,23.11
  Top 0.305: IC1.24 26.92,23.11 | 26.29,23.11 v24.77,21.59
  Top 0.61: R28.1 R29.2 23.28,11.01 v23.5,11.43
  Bottom 0.406: v23.5,11.43 23.5,20.32 v24.77,21.59
UVLO
  Top 0.305: 16.93,13.97 R3.1 R4.2 | 16.93,13.97 C2.2 | U3.7 16.8,14.11 16.93,13.97
VBATT  (via drill 0.5)
  Top 0.254: U3.5 11.06,13.61
  Top 0.305: 8.76,6.57 U2.3 | C10.1 8.76,5.08 | R3.2 18.63,13.97 | 18.63,13.97 C2.1 | v17.78,13.97 18.63,13.97
  Top 0.406: 11.06,13.61 10.16,12.7 9.29,12.7 L1.P$2
  Top 0.61: L1.P$2 7.85,13.11 v7.62,13.34 6.35,13.34 | 6.35,12.06 6.35,13.34 | 6.35,13.34 R2.1 | P4_PWRSW2.1 6.35,12.06 | 6.35,12.06 6.35,7.62 7.3,6.67 U2.3 | C1.1 8.76,5.08 8.76,6.57
  Bottom 0.406: v7.62,13.34 17.14,13.34 v17.78,13.97
VBUS
  Top 0.305: F1.2 23.88,6.73 24.1,6.51 U$2.1
VCAP1
  Top 0.305: IC1.31 33.58,19.61 32.38,18.41 C6.1
VCAP2
  Top 0.305: IC1.47 43.89,15.38 C7.1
